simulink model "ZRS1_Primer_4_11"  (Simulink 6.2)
settings: Solver=ode45  StartTime=0.0  StopTime=30  MaxStep=1  RelTol=1e-5
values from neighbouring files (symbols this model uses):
  k = 2    [basic_control.m]    (also in basic_control_1.m; ZRS1_Primer4_11.m = 0.7; ZRS1_Primer4_11_1.m = 0.7; ZRS2_primer_2_13.m = 100)
libraries: simulink x1

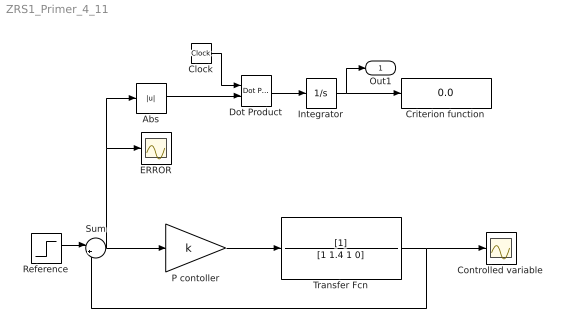
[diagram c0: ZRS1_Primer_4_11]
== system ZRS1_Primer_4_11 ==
  Abs : Abs
  Clock : Clock
  Controlled variable : Scope
  Criterion function : Display
  Dot Product : simulink/Math Operations/Dot Product  InputSameDT=on  OutDataType=sfix(16)  OutScaling=2^-10  DoSatur=off
  ERROR : Scope
  Integrator : Integrator
  P contoller : Gain  Gain=k
  Reference : Step  Time=0  SampleTime=0
  Sum : Sum  Inputs=|+-
  Transfer Fcn : TransferFcn  Denominator=[1 1.4 1 0]
  Out1 : Outport
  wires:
  Reference/1 -> Sum/1
  Sum/1 -> ERROR/1, Abs/1, P contoller/1
  Abs/1 -> Dot Product/2
  Clock/1 -> Dot Product/1
  Integrator/1 -> Criterion function/1, Out1/1
  Transfer Fcn/1 -> Controlled variable/1, Sum/2
  P contoller/1 -> Transfer Fcn/1
  Dot Product/1 -> Integrator/1
